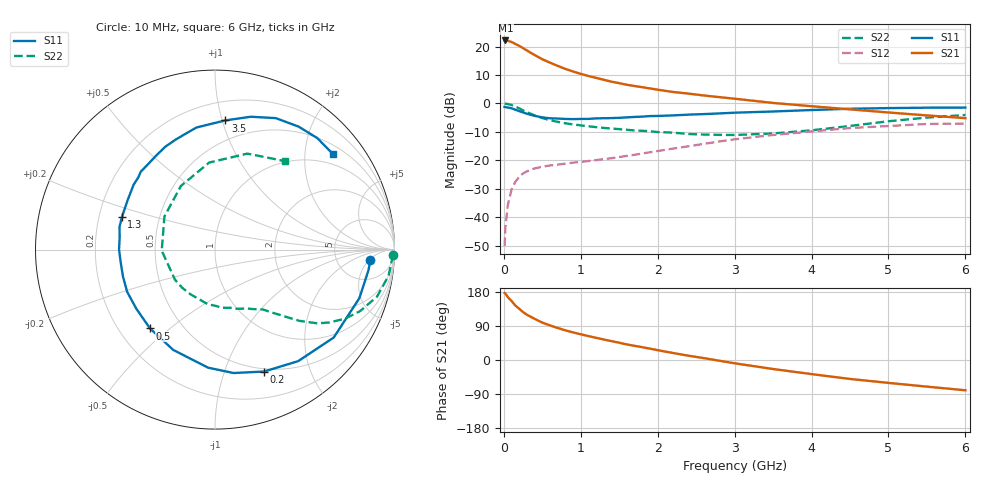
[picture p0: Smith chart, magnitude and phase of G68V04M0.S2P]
! SIEMENS Small Signal Semiconductors
! BFG193
! Si NPN RF Bipolar Junction Transistor in SOT223
! VCE = 8 V  IC = 4 mA
! Common Emitter S-Parameters:  August  1996
# GHz  S  MA  R  50
!  f  S11  S21  S12  S22
! GHz  MAG  ANG  MAG  ANG  MAG  ANG  MAG  ANG
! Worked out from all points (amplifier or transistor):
!   36 points, 10 MHz to 6 GHz, reference 50 ohm
!   highest |S21| = 22.1 dB at 20 MHz (marker M1)
!   |S21| within 3 dB of that: start of sweep to 268.5 MHz
!   unconditionally stable (mu >= 1): 1.225 GHz to 2.53 GHz
!   at 250 MHz: K = 0.28, MSG = 22.0 dB, |S12| = -24.6 dB
!   at 1.4 GHz: K = 1.08, MAG = 11.7 dB, |S12| = -19.3 dB
!   at 6 GHz: K = 0.88, MSG = 1.0 dB, |S12| = -7.1 dB
!   S11 on the Smith chart (normalised r, x): 10 MHz: 11, -6; 200 MHz: 0.47, -1.37; 500 MHz: 0.33, -0.43; 1.3 GHz: 0.30, +0.15; 3.5 GHz: 0.34, +1.02; 6 GHz: 0.71, +2.65
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0.01  0.8678 -4.0  12.79 177.0  0.0031 92.9  0.9932 -1.7
0.02  0.8626 -7.7  12.8 175.4  0.0065 88.1  0.9873 -3.4
0.05  0.8487 -18.6  12.61 166.4  0.016 78.8  0.9782 -8.5
0.1  0.8231 -36.5  12.05 155.7  0.0305 72.2  0.94 -16.2
0.15  0.7752 -53.3  11.11 143.7  0.0421 62.4  0.8779 -23.0
0.2  0.7322 -68.1  10.28 135.1  0.0513 56.7  0.8201 -28.0
0.25  0.6955 -81.4  9.394 126.4  0.0589 51.4  0.7553 -32.5
0.3  0.6592 -93.3  8.53 119.5  0.064 47.6  0.7044 -35.7
0.4  0.6054 -112.6  7.101 108.6  0.0721 41.7  0.6168 -40.1
0.5  0.5692 -129.5  5.985 98.7  0.0773 37.7  0.5534 -43.0
0.6  0.5484 -143.0  5.212 91.2  0.0813 35.8  0.5092 -45.4
0.7  0.5431 -154.3  4.578 84.5  0.0842 35.2  0.4755 -47.7
0.8  0.5343 -163.6  4.045 78.3  0.0873 34.3  0.4476 -49.7
1.1  0.5356 172.7  3.038 63.1  0.0972 35.2  0.3969 -56.7
1.3  0.5496 160.8  2.605 54.1  0.1052 36.2  0.3713 -61.8
1.6  0.5692 145.3  2.128 41.0  0.12 36.8  0.3449 -72.1
2.2  0.6165 122.5  1.591 18.5  0.1609 34.8  0.3074 -97.3
2.8  0.6676 103.8  1.292 -1.9  0.2146 27.5  0.2804 -130.9
3.5  0.7222 85.4  1.021 -23.8  0.279 13.3  0.2969 -178.8
4.5  0.807 65.2  0.787 -50.0  0.3695 -7.9  0.4024 118.1
5.5  0.843 47.5  0.616 -70.3  0.4357 -34.9  0.5642 71.4
6  0.8457 39.1  0.552 -79.9  0.4433 -50.1  0.6277 51.8
